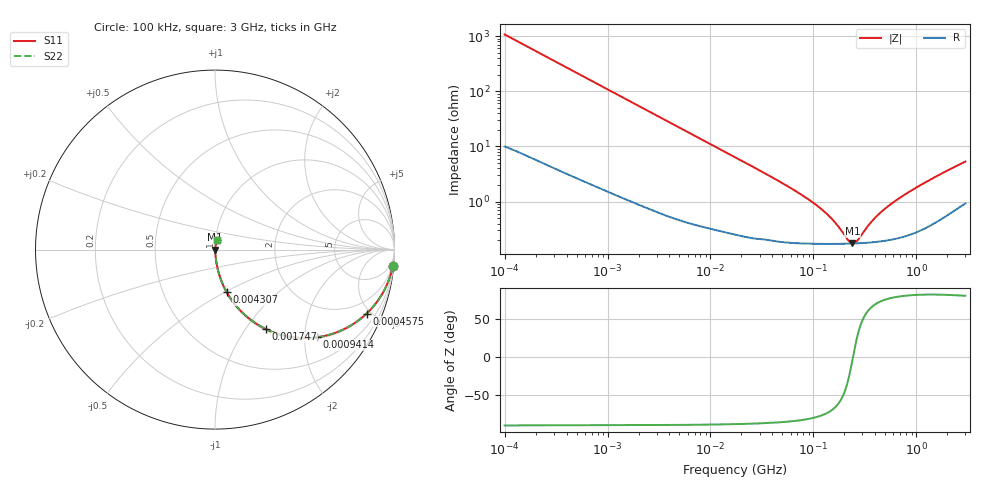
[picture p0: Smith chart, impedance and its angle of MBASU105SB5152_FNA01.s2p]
! MBASU105SB5152_FNA01  S-PARAMETER MODEL  ( Standard Model )
! Model Generated by TAIYO YUDEN Corporation (http://www.ty-top.com)
! Version 1.0
! TAIYO YUDEN Control No. 220601
! Copyright(c) 2013 TAIYO YUDEN CO.,LTD. All Rights Reserved.
! Product Description (link to TY-COMPAS)
! https://ds.yuden.co.jp/TYCOMPAS/or/detail?pn=MBASU105SB5152KFNA01&u=M
! Products Name : Multilayer Ceramic Capacitors
! Characteristics :
!  Capacitance : 1500 [pF] , Rated Voltage : 50 [V] , TCC : X5R
!  Case Size : 1.0 x 0.5 / 0.039 x 0.02 [mm/inch] , Thickness : 0.5 / 0.02 [mm/inch]
!  (Conditions: Temperature = 25 [degC] , DC Bias Voltage = 0 [V])
! External Node Assignments :
!  1  o---| |---o  2
! GND o---------o GND
! Frequency Range : 100kHz  -  3GHz  [ 401 STEP ]
# MHZ S RI R 50
! Freq[MHz].  S11 Real  S11 Imag  S21 Real  S21 Imag  S12 Real  S12 Imag  S22 Real  S22 Imag
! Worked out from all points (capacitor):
!   401 points, 100 kHz to 3 GHz, reference 50 ohm
!   read as one part in series: C = 1.49 nF near 105.3 kHz
!   lowest |Z| = 174 mohm at 240 MHz (marker M1)
!   series resonance near 242.9 MHz, so ESL is about 290 pH
!   S11 on the Smith chart (normalised r, x): 100 kHz: 1, -21; 457.5 kHz: 1.06, -4.71; 941.4 kHz: 1.03, -2.30; 1.747 MHz: 1.02, -1.25; 4.307 MHz: 1.01, -0.51; 3 GHz: 1.02, +0.10
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0.1  0.9904 -0.0928  0.00956 0.0928  0.00956 0.0928  0.9904 -0.0928
0.246461  0.9478 -0.217  0.0522 0.217  0.0522 0.217  0.9478 -0.217
0.457483  0.8445 -0.3564  0.1555 0.3564  0.1555 0.3564  0.8445 -0.3564
0.562235  0.7838 -0.4054  0.2162 0.4054  0.2162 0.4054  0.7838 -0.4054
0.941399  0.5693 -0.4883  0.4307 0.4883  0.4307 0.4883  0.5693 -0.4883
1.282589  0.4192 -0.4862  0.5808 0.4862  0.5808 0.4862  0.4192 -0.4862
1.747435  0.2831 -0.4428  0.7169 0.4428  0.7169 0.4428  0.2831 -0.4428
3.161081  0.1116 -0.306  0.8884 0.306  0.8884 0.306  0.1116 -0.306
4.306746  0.0652 -0.2372  0.9348 0.2372  0.9348 0.2372  0.0652 -0.2372
8.417093  0.0202 -0.128  0.9798 0.128  0.9798 0.128  0.0202 -0.128
17.7727  0.00633 -0.0618  0.9937 0.0618  0.9937 0.0618  0.00633 -0.0618
51.12795  0.00227 -0.0209  0.9977 0.0209  0.9977 0.0209  0.00227 -0.0209
97.38194  0.00182 -0.00966  0.9982 0.00966  0.9982 0.00966  0.00182 -0.00966
147.0833  0.00173 -0.00483  0.9983 0.00483  0.9983 0.00483  0.00173 -0.00483
171.6802  0.00172 -0.00327  0.9983 0.00327  0.9983 0.00327  0.00172 -0.00327
216.4987  0.00173 -0.00106  0.9983 0.00106  0.9983 0.00106  0.00173 -0.00106
240.0085  0.00174 -0.00011  0.9983 0.00011  0.9983 0.00011  0.00174 -0.00011
266.0711  0.00175 0.000843  0.9982 -0.000843  0.9982 -0.000843  0.00175 0.000843
381.6779  0.00185 0.00431  0.9981 -0.00431  0.9981 -0.00431  0.00185 0.00431
547.5153  0.00208 0.00833  0.9979 -0.00833  0.9979 -0.00833  0.00208 0.00833
1156.079  0.00354 0.0206  0.9965 -0.0206  0.9965 -0.0206  0.00354 0.0206
3000  0.0118 0.0513  0.9882 -0.0513  0.9882 -0.0513  0.0118 0.0513
